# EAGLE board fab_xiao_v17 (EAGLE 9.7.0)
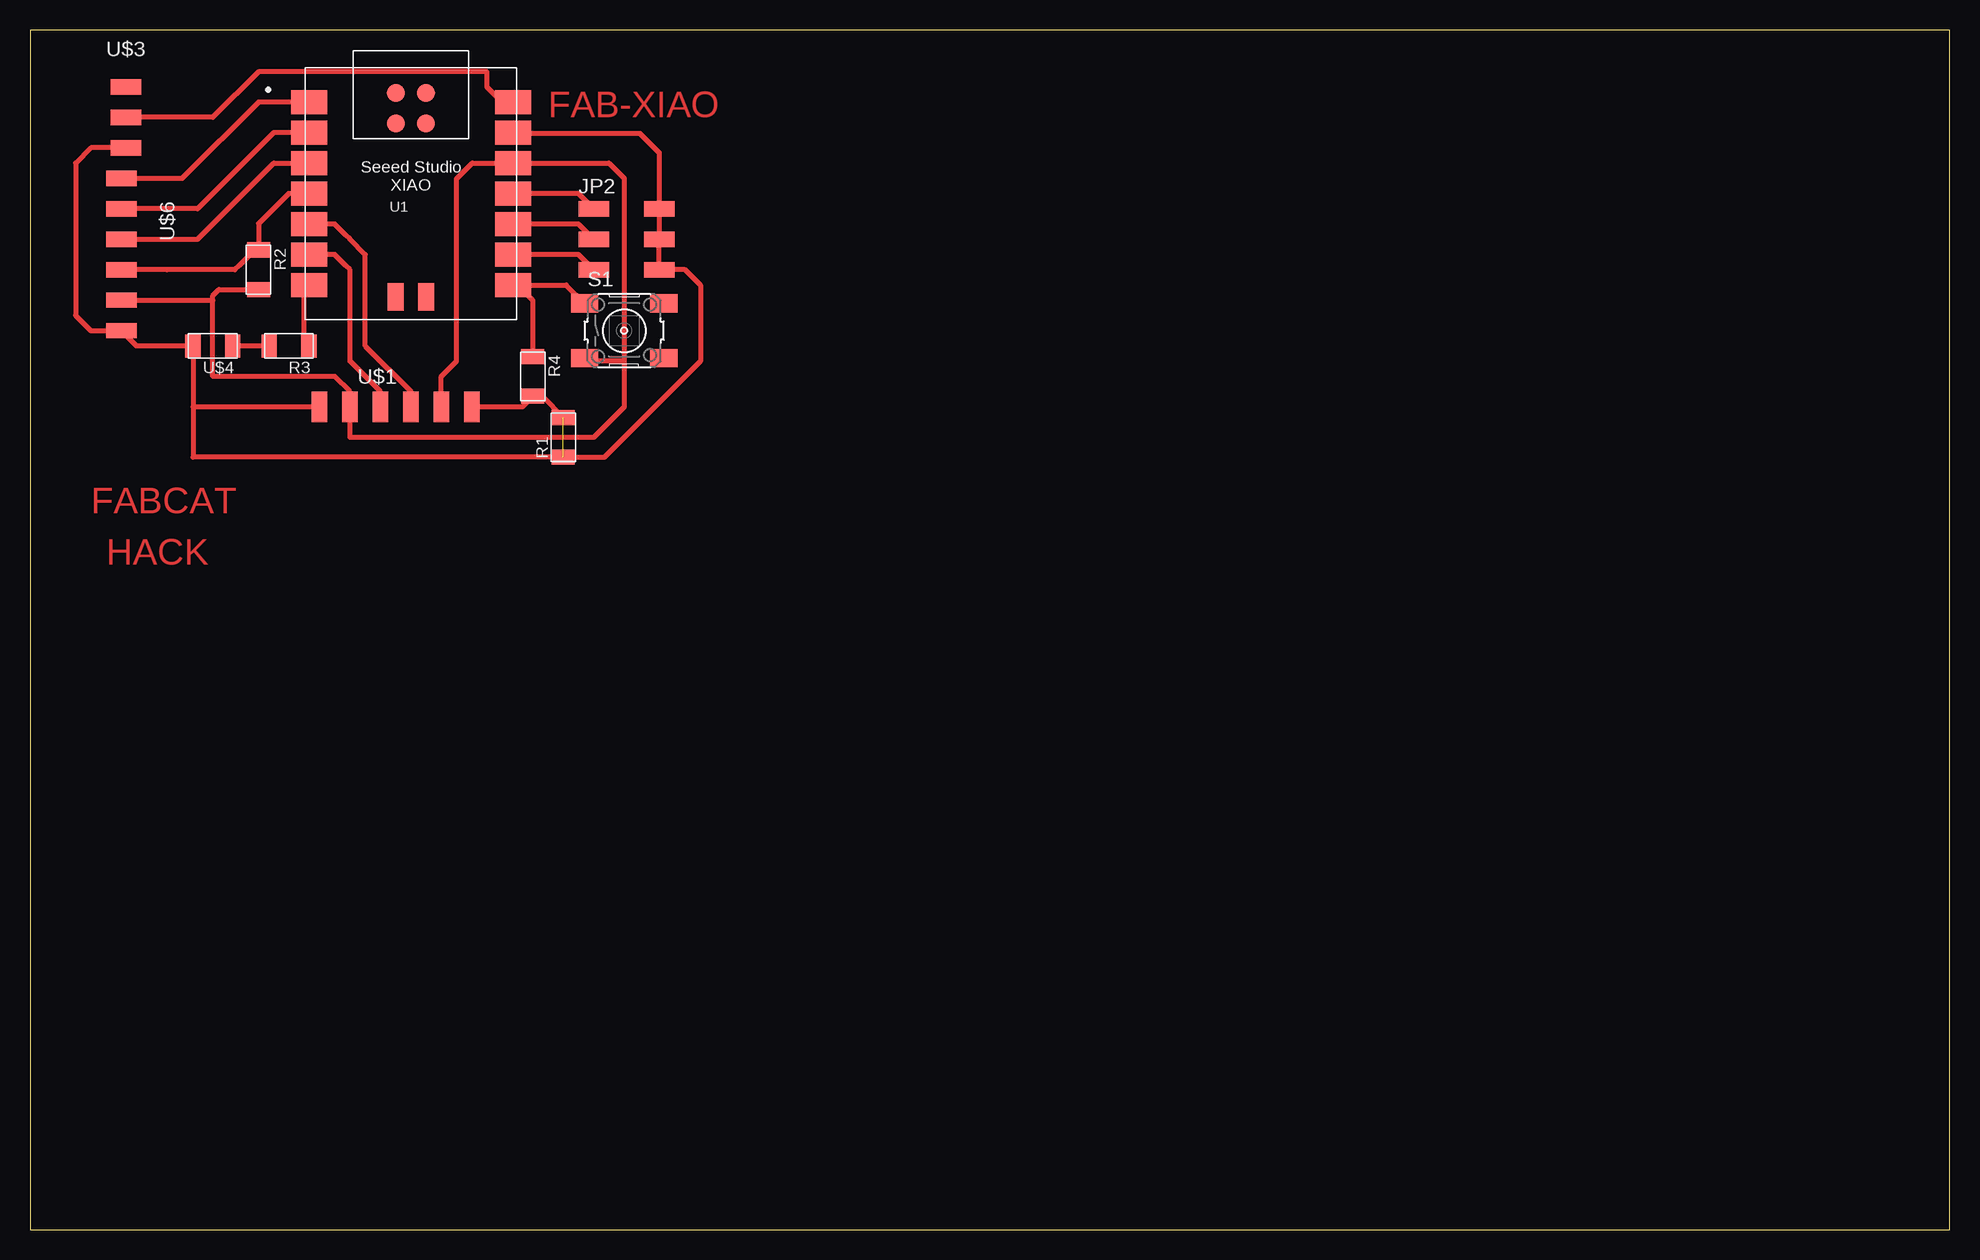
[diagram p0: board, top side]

Size 160 x 100 mm. Coordinates in mm from the lower left corner, seen from the top.
Outline: 0,0 160,0 160,100 0,100 0,0
Copper layers (1*16): Top 0.035mm / dielectric 1.5mm / Bottom 0.035mm
Design rules "default *": minimum track width 16mil, minimum drill 0.35mm, track to track 16mil, track to pad 16mil, pad to pad 16mil, via to via 16mil, smd to smd 6mil, copper to edge 40mil, drill to drill 6mil, minimum pad ring 10mil, minimum via ring 8mil, stop-mask expansion 4mil, vias tented up to drill 0mil, thermal gap 10mil

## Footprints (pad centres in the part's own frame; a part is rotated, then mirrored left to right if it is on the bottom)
2X03SMD = smd 2.54 x 1.27: 1 -2.54,2.54; 2 2.92,2.54; 3 -2.54,0; 4 2.92,0; 5 -2.54,-2.54; 6 2.92,-2.54
R1206FAB = smd 1.27 x 1.905: 1 -1.651,0; 2 1.651,0
6MM_SWITCH = smd 2.286 x 1.524: 1 -3.302,2.286; 2 3.302,2.286; 3 -3.302,-2.286; 4 3.302,-2.286
XIAO-SAMD21/RP2040-MODULE14P-2.54-21X17.8MM = smd 3 x 2: 1 -8.5,7.62; 2 -8.5,5.08; 3 -8.5,2.54; 4 -8.5,0; 5 -8.5,-2.54; 6 -8.5,-5.08; 7 -8.5,-7.62; 8 8.5,-7.62; 9 8.5,-5.08; 10 8.5,-2.54; 11 8.5,0; 12 8.5,2.54; 13 8.5,5.08; 14 8.5,7.62 | smd 1.5 x 1.5: 15 -1.27,8.39; 16 1.27,8.39; 17 -1.27,5.85; 18 1.27,5.85 | smd 1.3 x 2.3: 19 -1.27,-8.6; 20 1.27,-8.6
1X06SMD = smd 2.54 x 1.27: 1 0,6.35; 2 0,3.81; 3 0,1.27; 4 0,-1.27; 5 0,-3.81; 6 0,-6.35
SPDTSWITCH = smd 2.54 x 1.27: 1 0.38,2.54; 2 0.38,0; 3 0.38,-2.54
LED1206FAB = smd 1.27 x 1.905: 1 -1.651,0; 2 1.651,0

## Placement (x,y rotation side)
JP2  [2X03SMD]  49.53,82.55 0 top
R1  0  [R1206FAB]  44.45,66.04 90 top
R2  4.7K  [R1206FAB]  19.05,80.01 270 top
R3  1K  [R1206FAB]  21.59,73.66 180 top
R4  470  [R1206FAB]  41.91,71.12 270 top
S1  [6MM_SWITCH]  49.53,74.93 0 top
U1  XIAO-RP2040  [XIAO-SAMD21/RP2040-MODULE14P-2.54-21X17.8MM]  31.75,86.36 0 top
U$1  CONN_06_FTDI-SMD-HEADER  [1X06SMD]  30.48,68.58 270 top
U$3  SPDTSWITCH  [SPDTSWITCH]  7.62,92.71 0 top
U$4  LEDFAB1206  [LED1206FAB]  15.24,73.66 180 top
U$6  CONN_06_FTDI-SMD-HEADER  [1X06SMD]  7.62,81.28 180 top

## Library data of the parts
JP2 R1-R4 S1 U$1 U$3 U$4 U$6 = fab
U1 = Seeed Studio XIAO Series

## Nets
3V3: R2.2 S1.3 U1.12 U$1.2 U$1.5 U$6.2
5V [New Class]: U1.14 U$3.2
A0: U1.1 U$6.6
A1: U1.2 U$6.5
A2: U1.3 U$6.4
A3: R2.1 U1.4 U$6.3
A6: R3.1 U1.7
A7: R4.1 S1.1 U1.8
A8: JP2.5 U1.9
A9: JP2.3 U1.10
A10: JP2.1 U1.11
GND: JP2.2 JP2.4 JP2.6 R1.1 R1.2 R4.2 U1.13 U$1.1 U$1.6 U$3.3 U$4.2 U$6.1
N$2: U$3.1
N$3: R3.2 U$4.1
SCL: U1.6 U$1.4
SDA: U1.5 U$1.3

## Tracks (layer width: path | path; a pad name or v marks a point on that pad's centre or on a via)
3V3
  Top 0.406: 49.53,72.39 46.48,72.39 S1.3 | 49.53,72.39 49.53,87.63 48.26,88.9 U1.12 36.86,88.9 35.56,87.6 35.56,72.39 34.29,71.12 U$1.2 | 49.53,72.39 49.53,68.58 46.99,66.04 26.67,66.04 U$1.5 26.67,69.85 25.4,71.12 15.24,71.12 15.24,77.47 | 15.24,77.47 15.24,77.85 15.75,78.36 R2.2 | U$6.2 15.24,77.47
5V
  Top 0.406: U$3.2 15.24,92.71 19.05,96.52 38.1,96.52 38.1,95.25 39.37,93.98 U1.14
A0
  Top 0.406: U1.1 19.05,93.98 12.7,87.63 U$6.6
A1
  Top 0.406: U1.2 20.32,91.44 13.97,85.09 U$6.5
A2
  Top 0.406: U$6.4 13.97,82.55 20.32,88.9 U1.3
A3
  Top 0.406: U1.4 21.55,86.36 19.05,83.86 R2.1 18.73,81.66 17.43,80.36 17.08,80.01 11.43,80.01 U$6.3
A6
  Top 0.406: R3.1 22.86,73.66 22.86,78.35 U1.7
A7
  Top 0.406: S1.1 44.7,78.74 40.64,78.74 | U1.8 40.64,78.74 | 40.64,78.74 41.91,77.47 R4.1
A8
  Top 0.406: 46.65,80.35 JP2.5 45.72,81.28 U1.9
A9
  Top 0.406: 46.65,82.89 JP2.3 45.72,83.82 U1.10
A10
  Top 0.406: 46.65,85.43 JP2.1 45.72,86.36 U1.11
GND  (1 unrouted)
  Top 0.406: U$1.1 41.02,68.58 R4.2 42.67,69.47 R1.2 | U$3.3 5.08,90.17 3.81,88.9 3.81,76.2 5.08,74.93 U$6.1 8.89,73.66 U$4.2 13.59,68.58 | U1.13 40.32,91.37 50.87,91.37 52.45,89.79 JP2.2 JP2.4 JP2.6 54.61,80.01 55.88,78.74 55.88,72.39 47.88,64.39 R1.1 13.59,64.39 13.59,68.58 | U$1.6 16.51,68.58 13.59,68.58
N$3
  Top 0.406: R3.2 U$4.1
SCL
  Top 0.406: U$1.4 29.21,69.85 26.67,72.39 26.67,80.01 26.33,80.35 25.4,81.28 U1.6
SDA
  Top 0.406: U$1.3 31.75,69.85 27.94,73.66 27.94,81.28 26.67,82.55 26.33,82.89 25.4,83.82 U1.5 22.86,83.82

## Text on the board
Top: FAB-XIAO | FABCAT | HACK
